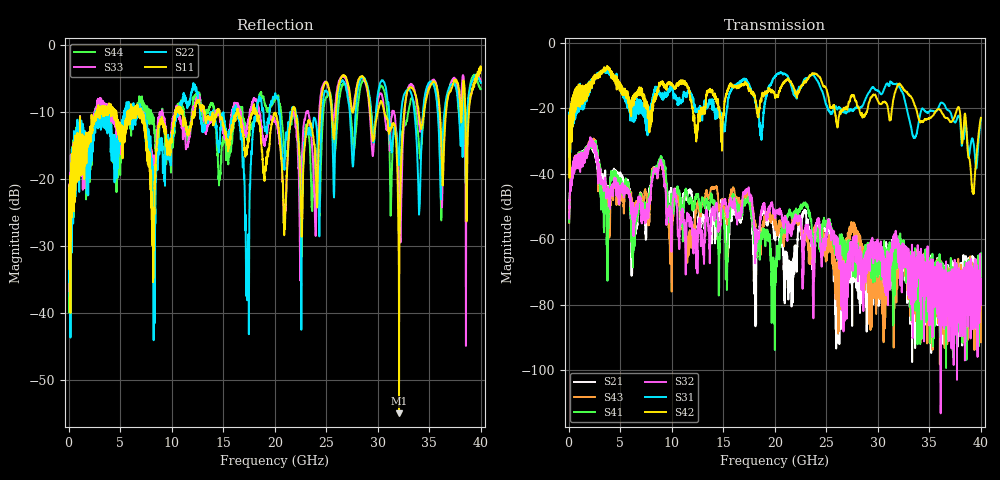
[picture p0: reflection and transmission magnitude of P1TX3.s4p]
!Agilent Technologies,N5245A,MY49151084,A.09.20.08
!Agilent N5245A: A.09.20.08
!Date: Thursday, March 01, 2012 14:47:08
!Correction: S11(Full 4 Port(1,2,3,4))
!S12(Full 4 Port(1,2,3,4))
!S13(Full 4 Port(1,2,3,4))
!S14(Full 4 Port(1,2,3,4))
!S21(Full 4 Port(1,2,3,4))
!S22(Full 4 Port(1,2,3,4))
!S23(Full 4 Port(1,2,3,4))
!S24(Full 4 Port(1,2,3,4))
!S31(Full 4 Port(1,2,3,4))
!S32(Full 4 Port(1,2,3,4))
!S33(Full 4 Port(1,2,3,4))
!S34(Full 4 Port(1,2,3,4))
!S41(Full 4 Port(1,2,3,4))
!S42(Full 4 Port(1,2,3,4))
!S43(Full 4 Port(1,2,3,4))
!S44(Full 4 Port(1,2,3,4))
!S4P File: Measurements: <S11,S12,S13,S14>,
!<S21,S22,S23,S24>,
!<S31,S32,S33,S34>,
!<S41,S42,S43,S44>:
# Hz S  dB  R 50
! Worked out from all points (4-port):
!   3996 points, 50 MHz to 40 GHz, reference 50 ohm
!   strongest paths, dB at 50 MHz, 10.04 GHz, 20.03 GHz, 30.02 GHz, 40 GHz:
!     S42: -26.5, -12.7, -16.6, -17.7, -22.9
!     S31: -25.2, -13.6, -10.3, -14.6, -23.2
!     S32: -53.7, -51.3, -53.0, -61.6, -78.0
!     S41: -54.8, -49.1, -68.6, -67.4, -64.3
!     S43: -55.0, -59.9, -54.5, -67.8, -91.5
!     S21: -54.7, -52.9, -59.4, -72.5, -70.9
!   lowest |S11| = -54.9 dB at 32.06 GHz (marker M1), VSWR 1.00, Z = 50 - j0.179 ohm
!   |S11| at or under -10 dB: start of sweep to 2.67 GHz; 7.083 GHz to 10.35 GHz (3.263 GHz wide, 37.4 % of centre); 18.22 GHz to 21.68 GHz (3.458 GHz wide, 17.3 % of centre)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
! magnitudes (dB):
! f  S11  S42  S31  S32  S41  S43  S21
! 50 MHz  -24.2  -26.5  -25.2  -53.7  -54.8  -55.0  -54.7
! 2.26 GHz  -12.5  -11.7  -11.7  -30.6  -31.6  -30.6  -31.5
! 6.27 GHz  -10.5  -18.5  -20.4  -54.3  -64.1  -51.5  -52.8
! 8.92 GHz  -11.2  -12.4  -15.7  -36.2  -35.2  -36.5  -35.9
! 19.87 GHz  -10.7  -14.7  -10.8  -51.8  -67.1  -52.4  -56.6
! 32.06 GHz  -54.9  -12.5  -13.4  -61.4  -61.1  -64.9  -64.0
! 40 GHz  -3.8  -22.9  -23.2  -78.0  -64.3  -91.5  -70.9
